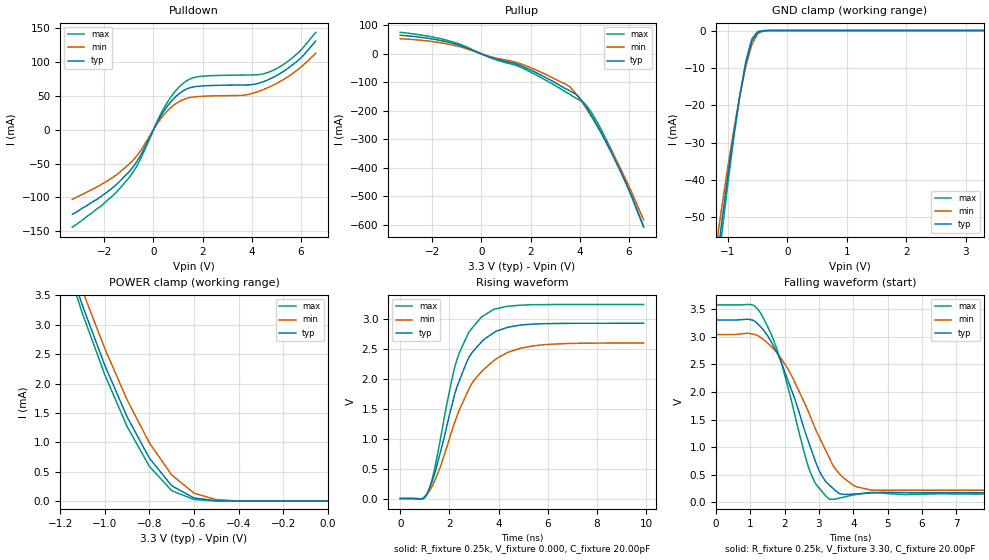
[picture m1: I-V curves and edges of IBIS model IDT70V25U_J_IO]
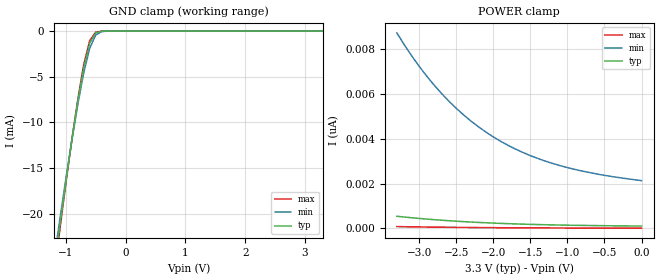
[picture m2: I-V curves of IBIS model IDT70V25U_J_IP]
| IBIS file 70v9359u.ibs created by s2ibis2 version 1.1
| North Carolina State University Electronics Research Laboratory  1995
[IBIS ver]   2.1
[File name]   70v9359u.ibs
[File Rev]   1.1
[Date]   10/30/01
[Source]   Integrated Device Technology, Inc.
[Notes]   1.Temperatures: typ=25C, min=0C, max=70C 2.Cemos9 process.
   3.Ramp rates based on 50 ohm load.
[Disclaimer] Integrated Device Technology, Inc. ("IDT") hereby grants the
   user of this IBIS model a non-exclusive, nontransferable
   license to use this IBIS model under the following terms. The
   user is granted this license only to use the IBIS model and is
   not granted rights to sell, copy (except as needed to run the
   IBIS model), rent, lease or sub-license the IBIS model in
   whole or in part, or in modified form to anyone. The User may
   modify the IBIS model to suit its specific applications, but
   rights to derivative works and such modifications shall belong
   to IDT. This IBIS model is provided on an AS IS" basis and IDT
   makes absolutely no warranty with respect to the information
   contained herein. IDT DISCLAIMS AND CUSTOMER WAIVES ALL
   WARRANTIES, EXPRESS AND IMPLIED, INCLUDING WARRANTIES OF
   MERCHANTABILITY AND FITNESS FOR A PARTICULAR PURPOSE. THE
   ENTIRE RISK AS TO QUALITY AND PERFORMANCE IS WITH THE USER
   ACCORDINGLY, IN NO EVENT SHALL IDT BE LIABLE FOR ANY DIRECT OR
   INDIRECT DAMAGES, WHETHER IN CONTRACT OR TORT, INCLUDING ANY
   LOST PROFITS OR OTHER INCIDENTAL, CONSEQUENTIAL, EXEMPLARY, OR
   PUNITIVE DAMAGES ARISING OUT OF THE USE OR APPLICATION OF THE
   IBIS model. Further, IDT reserves the right to make changes
   without notice to any product herein to improve reliability,
   function, or design. IDT does not convey any license under
   patent rights or any other intellectual property rights,
   including those of third parties. IDT is not obligated to
   provide maintenance or support for the licensed IBIS model.
[Copyright]   Copyright 2001, Integrated Device Technology, Inc. all rights
   reserved
|   Component 70v9359u
[Component]   70v9359u
[Manufacturer]   Integrated Device Technology
[Package]	 TQFP(PN100)
| variable   typ   min   max
R_pkg   10.00m   9.00m   11.00m
L_pkg   4.50nH   4.10nH   5.10nH
C_pkg   0.16pF   0.11pF   0.22pF
[Pin]  signal_name   model_name   R_pin   L_pin   C_pin
1	 A9L   IDT70V25U_J_IP
2	 A10L   IDT70V25U_J_IP
3	 A11L   IDT70V25U_J_IP
4	 A12L   IDT70V25U_J_IP
5   NC   NC
6   NC   NC
7   NC   NC
8	 LBL#   IDT70V25U_J_IP
9	 UBL#   IDT70V25U_J_IP
10   CE0L#   IDT70V25U_J_IP
11   CE1L   IDT70V25U_J_IP
12   CNTRRSTL#   IDT70V25U_J_IP
13   RWL   IDT70V25U_J_IP
14   OEL#   IDT70V25U_J_IP
15   VCC   POWER
16   FTPLL   IDT70V25U_J_IP
17   IO17L   IDT70V25U_J_IO
18   IO16L   IDT70V25U_J_IO
19   GND   GND
20   IO15L   IDT70V25U_J_IO
21   IO14L   IDT70V25U_J_IO
22   IO13L   IDT70V25U_J_IO
23   IO12L   IDT70V25U_J_IO
24   IO11L   IDT70V25U_J_IO
25   IO10L   IDT70V25U_J_IO
26   IO9L   IDT70V25U_J_IO
27   IO8L   IDT70V25U_J_IO
28   VCC   POWER
29   IO7L   IDT70V25U_J_IO
30   IO6L   IDT70V25U_J_IO
31   IO5L   IDT70V25U_J_IO
32   IO4L   IDT70V25U_J_IO
33   IO3L   IDT70V25U_J_IO
34   IO2L   IDT70V25U_J_IO
35   GND   GND
36   IO1L   IDT70V25U_J_IO
37   IO0L   IDT70V25U_J_IO
38   GND   GND
39   IO0R   IDT70V25U_J_IO
40   IO1R   IDT70V25U_J_IO
41   IO2R   IDT70V25U_J_IO
42   IO3R   IDT70V25U_J_IO
43   IO4R   IDT70V25U_J_IO
44   IO5R   IDT70V25U_J_IO
45   IO6R   IDT70V25U_J_IO
46   VCC   POWER
47   IO7R   IDT70V25U_J_IO
48   IO8R   IDT70V25U_J_IO
49   IO9R   IDT70V25U_J_IO
50   IO10R   IDT70V25U_J_IO
51   IO11R   IDT70V25U_J_IO
52   IO12R   IDT70V25U_J_IO
53   IO13R   IDT70V25U_J_IO
54   IO14R   IDT70V25U_J_IO
55   IO15R   IDT70V25U_J_IO
56   IO16R   IDT70V25U_J_IO
57   GND   GND
58   IO17R   IDT70V25U_J_IO
59   FTPLR   IDT70V25U_J_IP
60   OER#   IDT70V25U_J_IP
61   GND   GND
62   RWR   IDT70V25U_J_IP
63   CNTRRSTR#   IDT70V25U_J_IP
64   CE1R   IDT70V25U_J_IP
65   CE0R#   IDT70V25U_J_IP
66	 UBR#   IDT70V25U_J_IP
67	 LBR#   IDT70V25U_J_IP
68   NC   NC
69   NC   NC
70   NC   NC
71	 A12R   IDT70V25U_J_IP
72	 A11R   IDT70V25U_J_IP
73	 A10R   IDT70V25U_J_IP
74	 A9R   IDT70V25U_J_IP
75	 A8R   IDT70V25U_J_IP
76	 A7R   IDT70V25U_J_IP
77	 A6R   IDT70V25U_J_IP
78	 A5R   IDT70V25U_J_IP
79	 A4R   IDT70V25U_J_IP
80	 A3R   IDT70V25U_J_IP
81	 A2R   IDT70V25U_J_IP
82	 A1R   IDT70V25U_J_IP
83	 A0R   IDT70V25U_J_IP
84   CNTENR#   IDT70V25U_J_IP
85   CLKR   IDT70V25U_J_IP
86   ADSR#   IDT70V25U_J_IP
87   GND   GND
88   GND   GND
89   ADSL#   IDT70V25U_J_IP
90   CLKL   IDT70V25U_J_IP
91   CNTENL#   IDT70V25U_J_IP
92	 A0L   IDT70V25U_J_IP
93	 A1L   IDT70V25U_J_IP
94	 A2L   IDT70V25U_J_IP
95	 A3L   IDT70V25U_J_IP
96	 A4L   IDT70V25U_J_IP
97	 A5L   IDT70V25U_J_IP
98	 A6L   IDT70V25U_J_IP
99	 A7L   IDT70V25U_J_IP
100	 A8L   IDT70V25U_J_IP
| Models and submodels in the file (2): IDT70V25U_J_IO (I/O), IDT70V25U_J_IP (Input)
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| in   in   dummy_model
| oel  oel   dummy_model
|   Model IDT70V25U_J_IO
[Model]   IDT70V25U_J_IO
Model_type   I/O
Polarity   Non-Inverting
Enable   Active-High
Vinl =  0.800V
Vinh =  2.000V
Vmeas =  1.500V
C_comp   3.00pF   NA   NA
[Temperature Range]   25.00   70.00   0.000
[Voltage Range]   3.30V   3.00V   3.60V
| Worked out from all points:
|   slope of the pulldown table from 0 to 0.495 V, typ, clamps not added: 15.8 ohm
|   slope of the pullup table from 0 to 0.495 V, typ, clamps not added: 32.5 ohm
|   GND clamp passes 1 mA (typ) near -0.52 V on its own axis
|   POWER clamp passes 1 mA (typ) near -0.84 V on its own axis
|   rising waveform, R_fixture 0.25k, V_fixture 0.000, C_fixture 20.00pF: 20-80 % time 1.26ns typ, 1.59ns min, 1.11ns max; typ from 0 V to 2.93 V
|   falling waveform, R_fixture 0.25k, V_fixture 3.30, C_fixture 20.00pF: 20-80 % time 1.06ns typ, 1.28ns min, 892ps max; typ from 3.3 V to 0.177 V
[Pulldown]
| voltage   I(typ)   I(min)   I(max)
-3.3V     -125mA     -103mA     -144mA
-2.1V     -97.7mA    -80.5mA    -112mA
-1V       -62.57mA   -51.3mA    -71.34mA
-600mV    -42.68mA   -34.91mA   -48.6mA
400mV     26.25mA    20.98mA    30.45mA
800mV     45.07mA    35.54mA    52.93mA
1.2V      57.3mA     44.43mA    68.34mA
1.9V      64.51mA    49.27mA    78.77mA
3.7V      66.22mA    51.19mA    80.84mA
4.7V      74.44mA    62.92mA    85.24mA
5.9V      103mA      89.69mA    114mA
6.6V      131mA      113mA      144mA
[Pullup]
| voltage   I(typ)   I(min)   I(max)
-3.3V     65.49mA    53.26mA    75.61mA
-1.5V     44.15mA    36.71mA    50.07mA
500mV     -15.35mA   -12.68mA   -17.66mA
1.4V      -35mA      -29.56mA   -40.14mA
3.4V      -121mA     -105mA     -132mA
3.8V      -139mA     -135mA     -153mA
4V        -155mA     -158mA     -163mA
4.3V      -192mA     -196mA     -184mA
4.9V      -282mA     -281mA     -270mA
5.7V      -421mA     -410mA     -414mA
6.1V      -499mA     -483mA     -495mA
6.6V      -607mA     -583mA     -608mA
[GND_clamp]
| voltage   I(typ)   I(min)   I(max)
-3.3V     -440mA     -381mA     -493mA
-1.2V     -63.78mA   -58.2mA    -68.29mA
-1.1V     -50.94mA   -47.02mA   -54.16mA
-1V       -38.83mA   -36.43mA   -40.86mA
-900mV    -27.6mA    -26.55mA   -28.57mA
-800mV    -17.45mA   -17.52mA   -17.55mA
-700mV    -8.835mA   -9.688mA   -8.361mA
-600mV    -2.846mA   -3.826mA   -2.316mA
-500mV    -434uA     -859uA     -269uA
-400mV    -37.17uA   -111uA     -17.45uA
-300mV    -2.305uA   -10.81uA   -781nA
3.3V      112pA      422nA      13.12pA
[POWER_clamp]
| voltage   I(typ)   I(min)   I(max)
-3.3V     39.41mA    36.71mA    41.29mA
-1.2V     4.461mA    4.656mA    4.363mA
-1.1V     3.329mA    3.58mA     3.192mA
-1V       2.313mA    2.598mA    2.152mA
-900mV    1.434mA    1.725mA    1.27mA
-800mV    731uA      991uA      591uA
-700mV    262uA      445uA      177uA
-600mV    54.13uA    135uA      27.76uA
-500mV    6.835uA    25.51uA    2.736uA
-400mV    672nA      3.612uA    205nA
0V        112pA      2.189nA    14.61pA
[Ramp]
| variable   typ   min   max
dV/dt_r   1.10/0.68n   0.93/0.89n   1.28/0.57n
dV/dt_f   1.45/0.93n   1.21/1.14n   1.65/0.73n
R_load = 50.00
[Rising Waveform]
R_fixture = 0.25k
V_fixture = 0.000
C_fixture = 20.00pF
R_dut = 100.00m
L_dut = 4.00nH
C_dut = 0.60pF
| time   V(typ)   V(min)   V(max)
0s        0V         0V         0V
900ps     -6.586mV   -3.393mV   -3.119mV
1.1ns     88.88mV    78.48mV    75.24mV
1.4ns     415mV      296mV      502mV
2.3ns     1.861V     1.373V     2.315V
2.8ns     2.367V     1.836V     2.787V
3.3ns     2.614V     2.118V     3.033V
4.3ns     2.852V     2.427V     3.209V
5.3ns     2.913V     2.544V     3.239V
9.9ns     2.93V      2.6V       3.243V
[Falling Waveform]
R_fixture = 0.25k
V_fixture = 3.30
C_fixture = 20.00pF
R_dut = 100.00m
L_dut = 4.00nH
C_dut = 0.60pF
| time   V(typ)   V(min)   V(max)
0s        3.3V       3.036V     3.572V
1ns       3.306V     3.054V     3.579V
1.3ns     3.176V     2.984V     3.424V
1.9ns     2.535V     2.602V     2.535V
2.7ns     1.09V      1.63V      626mV
3ns       582mV      1.192V     264mV
3.3ns     317mV      808mV      58.32mV
3.7ns     148mV      453mV      93.98mV
4.5ns     172mV      226mV      180mV
9.9ns     177mV      220mV      153mV
|   Model IDT70V25U_J_IP
[Model]   IDT70V25U_J_IP
Model_type   Input
Vinl =  0.800V
Vinh =  2.000V
Vmeas =  1.500V
C_comp   3.00pF   NA   NA
[Temperature Range]   25.00   70.00   0.000
[Voltage Range]   3.30V   3.00V   3.60V
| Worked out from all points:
|   GND clamp passes 1 mA (typ) near -0.57 V on its own axis
[GND_clamp]
| voltage   I(typ)   I(min)   I(max)
-3.3V     -143mA     -134mA     -148mA
-1.2V     -26.3mA    -25.2mA    -26.99mA
-1.1V     -21.34mA   -20.64mA   -21.78mA
-1V       -16.55mA   -16.23mA   -16.74mA
-900mV    -11.98mA   -12.02mA   -11.94mA
-800mV    -7.724mA   -8.076mA   -7.493mA
-700mV    -4.012mA   -4.576mA   -3.659mA
-600mV    -1.336mA   -1.876mA   -1.039mA
-500mV    -206uA     -436uA     -119uA
-400mV    -17.54uA   -56.87uA   -7.617uA
-300mV    -1.075uA   -5.505uA   -337nA
3.3V      109pA      2.266nA    13.01pA
[POWER_clamp]
| voltage   I(typ)   I(min)   I(max)
-3.3V     545pA      8.718nA    84.03pA
-3.2V     510pA      8.189nA    78.64pA
-3V       448pA      7.232nA    68.83pA
-2.7V     369pA      6.027nA    56.34pA
-2.4V     305pA      5.062nA    46.2pA
-2.2V     270pA      4.534nA    40.57pA
-2V       240pA      4.085nA    35.73pA
-1.8V     215pA      3.706nA    31.59pA
-1.6V     193pA      3.388nA    28.07pA
-1.2V     160pA      2.9nA      22.58pA
-700mV    132pA      2.491nA    17.95pA
0V        109pA      2.133nA    14.11pA
